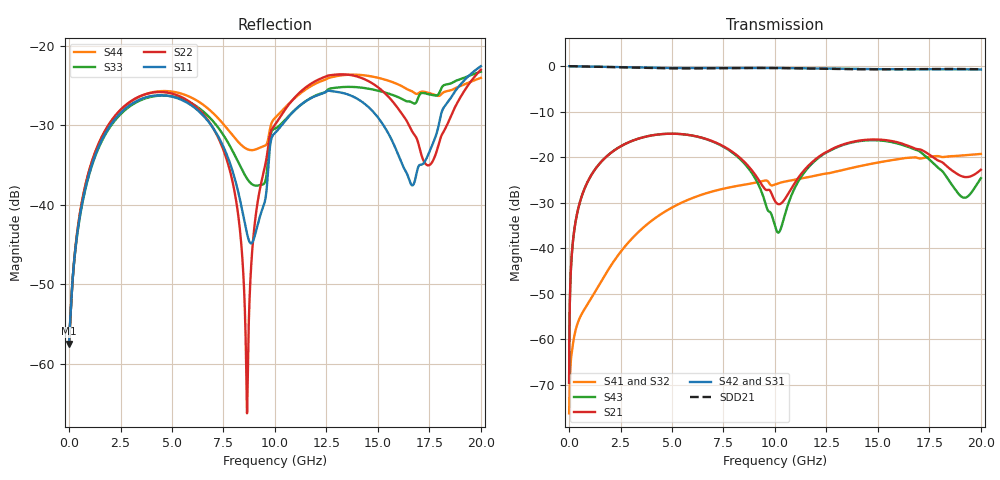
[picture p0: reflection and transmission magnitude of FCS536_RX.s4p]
!Generated from:
! 1
! 2
! 3
! 4
!PowerSI Version: 17.0.2.03131.86335  002
!Computer Host Name: W764D-PINDIS
!TouchstoneFormatFlag = 1
! GNDNET
! NETSLIST
!User Comments:
!  Touchstone file from project M5P200_FCS536_071117_85Ohm_112717
!  Exported from HFSS 3D Layout Design 2017.2.0
!  Port[1] = BGA.G30.SERDES_0_RX0_N
!  Port[2] = BGA.H30.SERDES_0_RX0_P
!  Port[3] = DIE1.400.SERDES_0_RX0_N
!  Port[4] = DIE1.401.SERDES_0_RX0_P
!  freq  S11mag  S11ang  S12mag
!  S12ang  S13mag  S13ang  S1
!  4mag  S14ang
!  S21mag  S21ang  S22mag
!  S22ang  S23mag  S23ang  S2
!  4mag  S24ang
!  S31mag  S31ang  S32mag
!  S32ang  S33mag  S33ang  S3
!  4mag  S34ang
!  S41mag  S41ang  S42mag
!  S42ang  S43mag  S43ang  S4
!  4mag  S44ang
#	Hz	S	RI	R	50
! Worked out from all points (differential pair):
!   4999 points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, 4.001 MHz to 20 GHz, reference 50 ohm
!   strongest paths, dB at 4.001 MHz, 5.001 GHz, 10 GHz, 15 GHz, 20 GHz:
!     S42: 0.0, -0.4, -0.4, -0.7, -0.7
!     S31: 0.0, -0.4, -0.4, -0.7, -0.8
!     S21: -69.5, -14.8, -29.6, -16.1, -22.8
!     S43: -69.5, -14.8, -35.1, -16.3, -24.6
!     S41: -76.3, -31.1, -26.0, -21.2, -19.3
!     S32: -76.3, -31.0, -26.0, -21.3, -19.4
!   taken as a pair (ports 2,1 in; 4,3 out), SDD21 dB: 0.0, -0.5, -0.4, -0.7, -0.7
!   lowest |S11| = -57.5 dB at 4.001 MHz (marker M1), VSWR 1.00, Z = 50.1 + j0.0126 ohm
!   |S11| at or under -10 dB: start of sweep to end of sweep
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4000800  0.00133 0.000126  0.000146 0.0003  0.9987 -0.00153  -0.000142 -5.93e-05
         0.000146 0.0003  0.00132 0.000117  -0.000142 -5.93e-05  0.9987 -0.00151
         0.9987 -0.00153  -0.000142 -5.93e-05  0.00133 0.000126  0.000146 0.0003
         -0.000142 -5.93e-05  0.9987 -0.00151  0.000146 0.0003  0.00132 0.000117
5.921184e8  0.00475 -0.00825  0.00785 0.0349  0.9728 -0.1924  -0.000869 -0.00164
            0.00785 0.0349  0.00453 -0.00882  -0.000854 -0.00163  0.9732 -0.1908
            0.9728 -0.1924  -0.000854 -0.00163  0.00481 -0.00805  0.00831 0.0348
            -0.000869 -0.00164  0.9732 -0.1908  0.00831 0.0348  0.00464 -0.00865
3.068614e9  -0.0283 -0.0328  0.1224 0.0887  0.5406 -0.8016  -0.00595 -0.0114
            0.1224 0.0887  -0.0304 -0.0337  -0.00609 -0.0114  0.5472 -0.7974
            0.5406 -0.8016  -0.00609 -0.0114  -0.0246 -0.0348  0.1289 0.0792
            -0.00595 -0.0114  0.5472 -0.7974  0.1289 0.0792  -0.0261 -0.0368
7.329466e9  -0.0244 0.00801  0.1206 -0.0666  -0.6246 -0.7191  -0.0371 0.0239
            0.1206 -0.0666  -0.0224 0.0111  -0.0367 0.0252  -0.611 -0.7316
            -0.6246 -0.7191  -0.0367 0.0252  -0.0294 -0.00215  0.0933 -0.0993
            -0.0371 0.0239  -0.611 -0.7316  0.0933 -0.0993  -0.0335 -0.00589
8.641728e9  -0.00654 -0.000865  0.062 -0.055  -0.8607 -0.4113  -0.0249 0.0439
            0.062 -0.055  -0.000392 -0.000291  -0.0231 0.0451  -0.8519 -0.4315
            -0.8607 -0.4113  -0.0231 0.0451  -0.0131 -0.00649  0.0202 -0.0763
            -0.0249 0.0439  -0.8519 -0.4315  0.0202 -0.0763  -0.0191 -0.0116
1.074215e10  -0.00841 -0.0358  0.0337 0.0272  -0.9284 0.1998  0.00686 0.0549
             0.0337 0.0272  -0.000733 -0.0438  0.00961 0.0538  -0.9345 0.1751
             -0.9284 0.1998  0.00961 0.0538  -0.00662 -0.0363  -0.00737 0.0345
             0.00686 0.0549  -0.9345 0.1751  -0.00737 0.0345  -0.0173 -0.0406
2e10  0.0346 -0.0659  0.0597 0.0415  0.9131 0.0445  0.0115 -0.1079
      0.0597 0.0415  0.0498 -0.0501  0.00286 -0.1074  0.9134 0.0922
      0.9131 0.0445  0.00286 -0.1074  -0.0163 -0.0668  -0.0425 0.0405
      0.0115 -0.1079  0.9134 0.0922  -0.0425 0.0405  -0.0358 -0.0516
